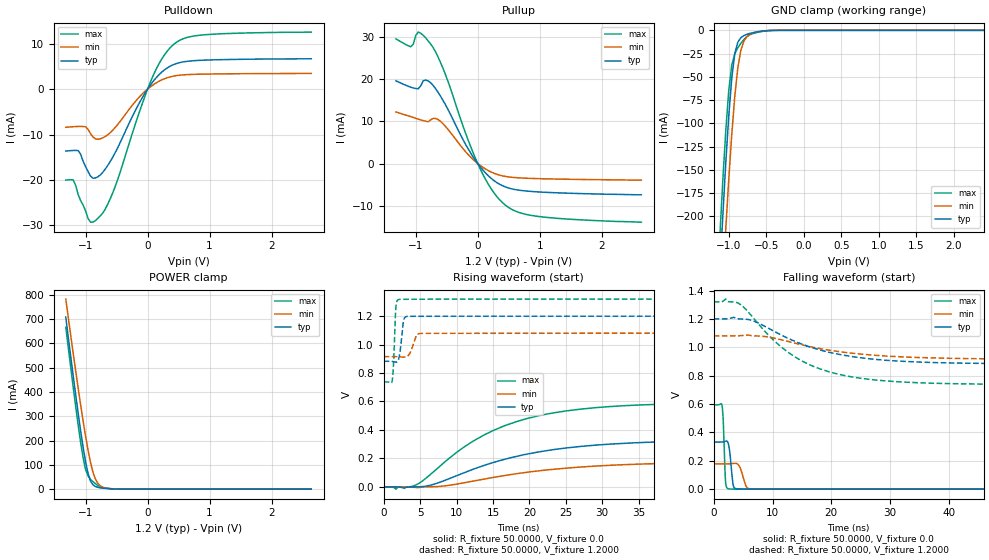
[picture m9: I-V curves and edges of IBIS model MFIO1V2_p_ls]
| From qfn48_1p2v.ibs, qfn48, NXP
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[Model] MFIO1V2_p_ls
|   Model MFIO1V2_p_ls
| This model was characterised for following simulation conditions:
| External (pad) voltage:
|   - Typ: 1.2V,   - Min: 1.08V,   - Max: 1.32V
| Library cells for typ/min/max conditions are connected as defined below:
|  IO - External Pad
|  A - Core Input
|  EN - Output Buffer Enable
|  BOOST - vdde
|  EHS - gnd
|  ENZI - vdd
|  EPD - gnd
|  EPUN - vdd
|  ZI - NC
|  ZIF - NC
|  gnd - gnd
|  gnde - gnde
|  vdd - vdd
|  vdde - vdde
| All other pins connected to ground
Model_type I/O
Polarity   Non-Inverting
Enable   Active-Low
Vinl =   0.3600V
Vinh =   0.8400V
Vmeas =  0.6000V
Cref =   20.0000F
Rref =   1.0000M
Vref =   0.0V
C_comp   1.6652pF   1.5787pF   1.7428pF
|C_comp_pullup   0.8462pF   0.8814pF   0.7990pF
|C_comp_pulldown   0.6044pF   0.6428pF   0.5687pF
[Model Spec]
| variable   typ   min   max
Vinh   0.3600V   0.3240V   0.3960V
Vinl   0.8400V   0.7560V   0.9240V
Vmeas   0.6000V   0.5400V   0.6600V
[Temperature Range]   25.0000   0.1250k   -40.0000
[Voltage Range]   1.2000V   1.0800V   1.3200V
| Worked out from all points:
|   slope of the pulldown table from 0 to 0.18 V, typ, clamps not added: 58.2 ohm
|   slope of the pullup table from 0 to 0.18 V, typ, clamps not added: 59.4 ohm
|   GND clamp passes 1 mA (typ) near -0.57 V on its own axis
|   POWER clamp passes 1 mA (typ) near -0.54 V on its own axis
|   rising waveform, R_fixture 50.0000, V_fixture 0.0: 20-80 % time 14.4ns typ, 16.1ns min, 12.2ns max; typ from 0 V to 0.332 V
|   rising waveform, R_fixture 50.0000, V_fixture 1.2000: 20-80 % time 406ps typ, 668ps min, 259ps max; typ from 0.883 V to 1.2 V
|   falling waveform, R_fixture 50.0000, V_fixture 0.0: 20-80 % time 465ps typ, 792ps min, 298ps max; typ from 0.332 V to 0 V
|   falling waveform, R_fixture 50.0000, V_fixture 1.2000: 20-80 % time 12.6ns typ, 13.9ns min, 10.9ns max; typ from 1.2 V to 0.883 V
[Pulldown]
|Voltage   I(typ)   I(min)   I(max)
-1.32V    -13.65mA   -8.413mA   -20.02mA
-1.2V     -13.51mA   -8.286mA   -20.01mA
-1.12V    -13.55mA   -8.228mA   -23.23mA
-920mV    -19.16mA   -9.849mA   -29.29mA
-720mV    -18.27mA   -10.7mA    -27.21mA
-520mV    -13.92mA   -8.406mA   -21.33mA
-160mV    -3.727mA   -2.148mA   -6.154mA
80mV      1.535mA    840.4uA    2.681mA
280mV     4.299mA    2.312mA    7.674mA
480mV     5.684mA    2.989mA    10.42mA
960mV     6.383mA    3.3mA      11.99mA
2.64V     6.671mA    3.446mA    12.53mA
[Pullup]
|Voltage   I(typ)   I(min)   I(max)
-1.32V    19.64mA    12.26mA    29.61mA
-1.08V    18.12mA    11.13mA    27.73mA
-960mV    17.74mA    10.54mA    31.21mA
-840mV    19.83mA    10.07mA    29.84mA
-720mV    18.57mA    10.71mA    27.56mA
-520mV    13.94mA    8.794mA    21.09mA
-200mV    4.663mA    2.883mA    7.362mA
40mV      -771.3uA   -452.7uA   -1.28mA
240mV     -3.804mA   -2.171mA   -6.507mA
480mV     -5.732mA   -3.143mA   -10.26mA
1.04V     -6.794mA   -3.614mA   -12.68mA
2.64V     -7.439mA   -3.951mA   -13.93mA
[GND_clamp]
|Voltage   I(typ)   I(min)   I(max)
-1.32V    -596.2mA   -647.7mA   -564.2mA
-1.12V    -261.7mA   -329.6mA   -222.8mA
-1.08V    -200.1mA   -270.2mA   -162.2mA
-1.04V    -142.4mA   -213.4mA   -108mA
-1V       -91.65mA   -160.1mA   -64.39mA
-960mV    -51.25mA   -111.8mA   -37.35mA
-920mV    -25.17mA   -71.04mA   -25.18mA
-880mV    -12.88mA   -40.68mA   -18.84mA
-800mV    -5.691mA   -11.78mA   -10.04mA
-680mV    -2.577mA   -2.919mA   -3.527mA
-440mV    -153.3uA   -179.9uA   -188.4uA
2.64V     0A         0A         0A
[POWER_clamp]
|Voltage   I(typ)   I(min)   I(max)
-1.32V    708.1mA    782.2mA    666.5mA
-1.2V     465.4mA    558mA      418.6mA
-1.12V    311.6mA    414.7mA    262.8mA
-1.04V    171.5mA    279.6mA    128mA
-1V       111.6mA    216.9mA    80.26mA
-960mV    64.04mA    159.3mA    53.83mA
-920mV    32.99mA    108.8mA    40.2mA
-880mV    17.4mA     68.42mA    30.38mA
-840mV    10.74mA    40.16mA    22.02mA
-760mV    5.263mA    13.19mA    9.321mA
-440mV    204.8uA    279.1uA    238.1uA
2.64V     0A         0A         0A
[Ramp]
| variable   typ   min   max
dV/dt_r  0.1990/14.4400n   0.1067/16.0908n   0.3564/12.2186n
dV/dt_f  0.1903/12.5923n   98.6839m/13.9393n   0.3495/10.8893n
R_load = 50.0000
[Rising Waveform]
R_fixture= 50.0000
V_fixture= 0.0
V_fixture_min= 0.0
V_fixture_max= 0.0
|time   V(typ)   V(min)   V(max)
0s        1.255nV    120.3nV    51.27pV
1.702ns   73.16uV    73.79uV    -16.42mV
4.457ns   -535.6uV   -4.409mV   13.58mV
6.761ns   15.97mV    389.6uV    102.1mV
10.98ns   97.92mV    27.72mV    277.9mV
16.64ns   193.9mV    79.97mV    430.5mV
21.31ns   245.7mV    112.5mV    500.3mV
26.62ns   281.8mV    137.8mV    544.2mV
45.12ns   324.5mV    170.8mV    588.2mV
100ns     331.7mV    177.8mV    594.1mV
[Rising Waveform]
R_fixture= 50.0000
V_fixture= 1.2000
V_fixture_min= 1.0800
V_fixture_max= 1.3200
|time   V(typ)   V(min)   V(max)
0s        882.9mV    915.5mV    737.5mV
1.165ns   881.5mV    915.7mV    743.7mV
1.361ns   879.5mV    915.8mV    865.6mV
1.678ns   876.3mV    915.1mV    1.262V
2.148ns   918.5mV    913.5mV    1.318V
2.745ns   1.17V      911.4mV    1.319V
3.308ns   1.198V     919.6mV    1.319V
4.551ns   1.199V     1.068V     1.319V
5.319ns   1.199V     1.079V     1.319V
100ns     1.2V       1.08V      1.32V
[Falling Waveform]
R_fixture= 50.0000
V_fixture= 0.0
V_fixture_min= 0.0
V_fixture_max= 0.0
|time   V(typ)   V(min)   V(max)
0s        331.7mV    177.8mV    594.1mV
1.411ns   332mV      177.8mV    588.3mV
1.612ns   333.7mV    177.7mV    478.9mV
2.003ns   338.2mV    177.6mV    53.46mV
2.543ns   309.7mV    178.5mV    1.864mV
3.295ns   30.92mV    181.5mV    944.3uV
4.019ns   1.274mV    177.8mV    942.9uV
5.54ns    648.3uV    17.1mV     623.3uV
6.555ns   570.9uV    1.068mV    454.2uV
100ns     11.3nV     162.5nV    8.903nV
[Falling Waveform]
R_fixture= 50.0000
V_fixture= 1.2000
V_fixture_min= 1.0800
V_fixture_max= 1.3200
|time   V(typ)   V(min)   V(max)
0s        1.2V       1.08V      1.32V
2.008ns   1.2V       1.08V      1.34V
4.425ns   1.2V       1.082V     1.306V
6.56ns    1.189V     1.081V     1.215V
10.26ns   1.113V     1.065V     1.046V
15.45ns   1.016V     1.013V     894.2mV
19.35ns   967.5mV    981.8mV    830.5mV
24.91ns   926.6mV    952.5mV    782.3mV
43.34ns   887.5mV    920.3mV    741.7mV
100ns     882.9mV    915.5mV    737.5mV
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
